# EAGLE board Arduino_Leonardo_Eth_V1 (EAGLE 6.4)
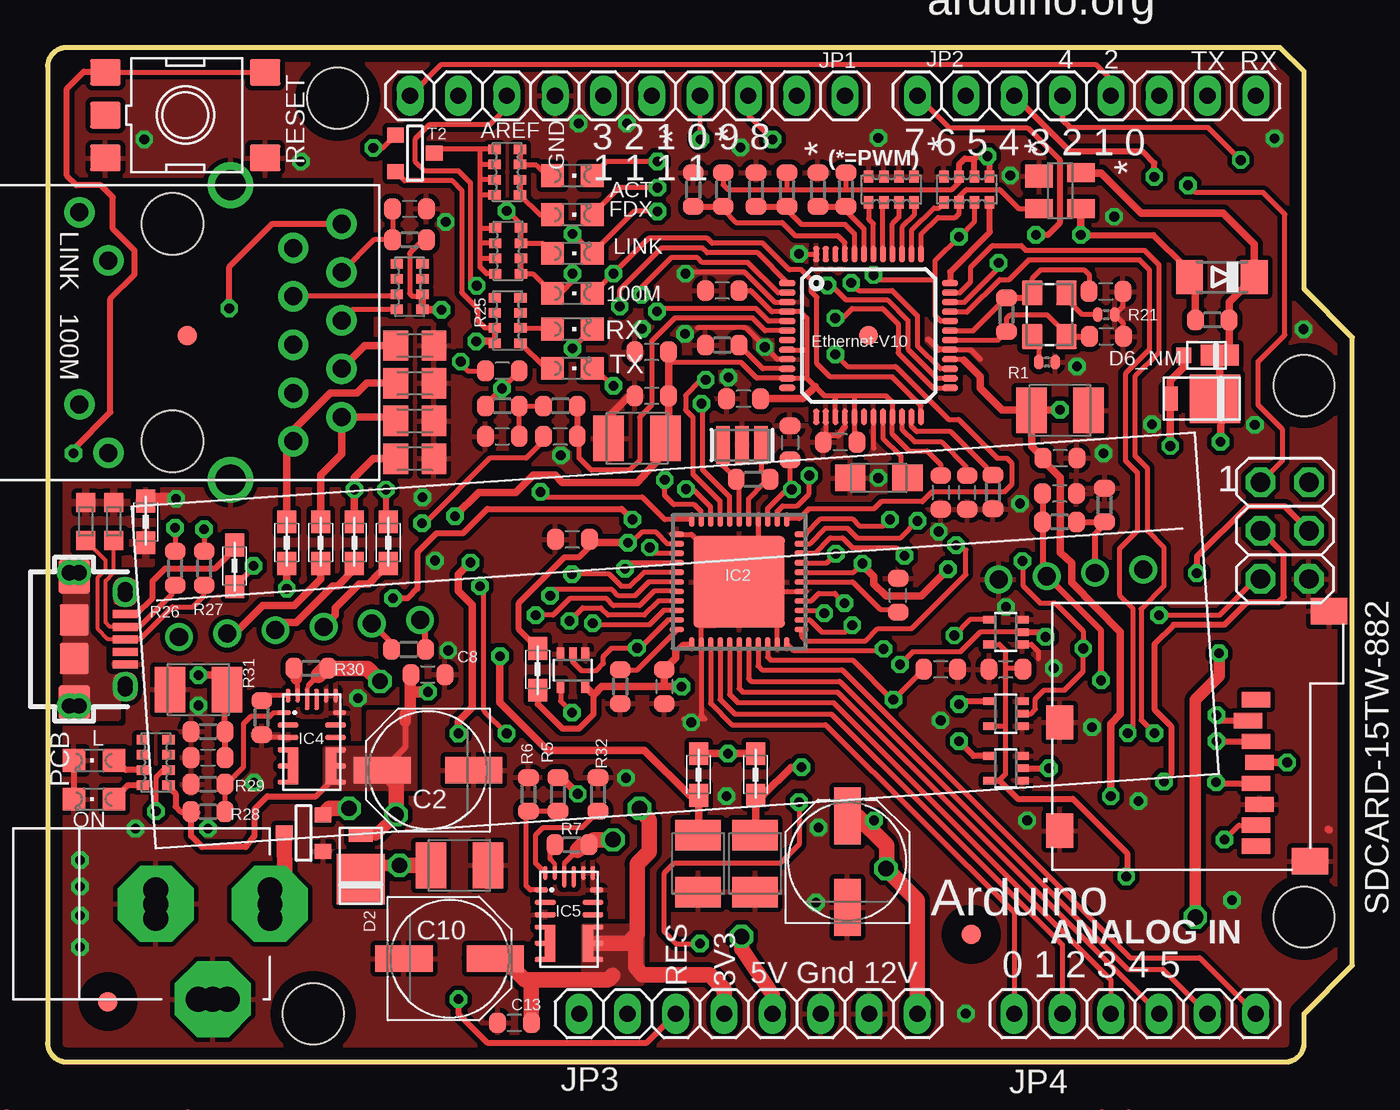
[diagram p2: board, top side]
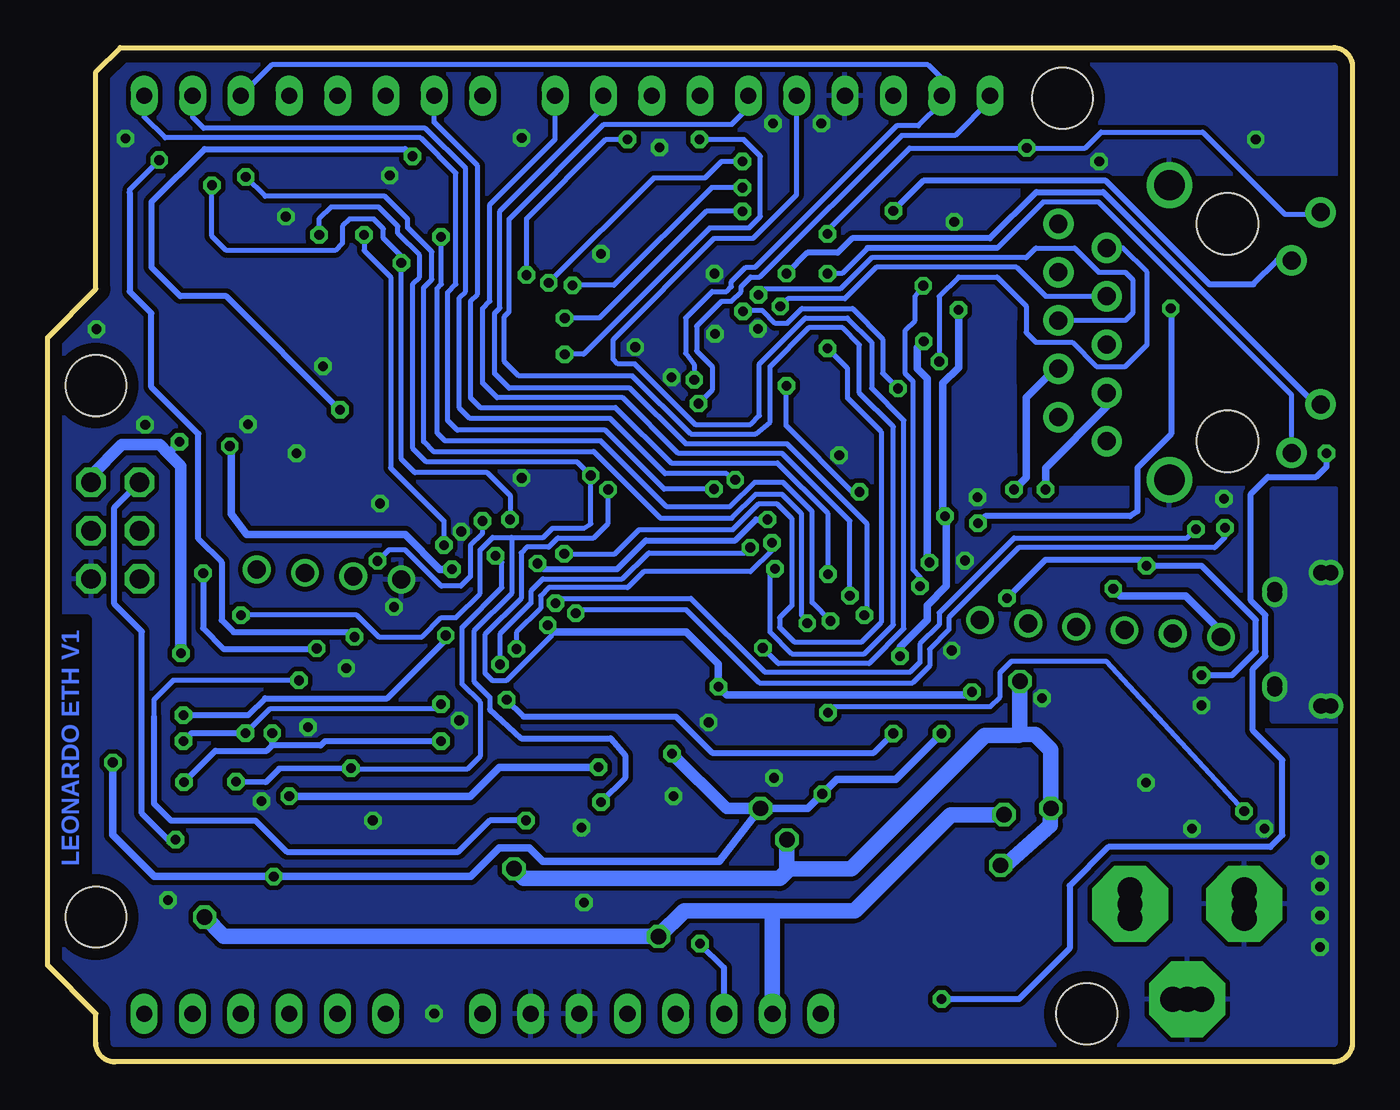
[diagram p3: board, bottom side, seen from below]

Size 68.58 x 53.34 mm. Coordinates in mm from the lower left corner, seen from the top.
Outline: 66.04,2.54 68.58,5.08 68.58,38.1 66.04,40.64 66.04,52.07 64.77,53.34 1,53.34 arc90 0,52.34 0,1 arc90 1,0 65.04,0 arc90 66.04,1 66.04,2.54
Copper layers (1*16): Top 0.035mm / dielectric 1.5mm / Bottom 0.035mm
Design rules "default *": minimum track width 10mil, minimum drill 20mil, track to track 8mil, track to pad 8mil, pad to pad 4mil, via to via 8mil, smd to smd 4mil, copper to edge 25mil, drill to drill 10mil, minimum pad ring 10mil, minimum via ring 8mil, stop-mask expansion 1mil, vias tented up to drill 33mil, thermal gap 10mil
Net classes: 0 default: width 0.254 mm, drill 0.508 mm, clearance 0.102 mm; 1 power: width 0.254 mm, drill 0.508 mm, clearance 0.203 mm; 2 gnd: width 0.254 mm, drill 0.508 mm, clearance 0.254 mm; 3 usbvcc: width 0.254 mm, drill 0.508 mm, clearance 0.254 mm; 4 aref: width 0.254 mm, drill 0.508 mm, clearance 0.203 mm; 5 ETH: width 0.305 mm, drill 0.508 mm, clearance 0.762 mm to class 0, clearance 0.762 mm to class 1, clearance 0.762 mm to class 2, clearance 0.762 mm to class 3, clearance 0.762 mm to class 4
Holes 3.2 mm at 66.04,35.56 66.04,7.62 15.24,50.67 13.97,2.54
bRestrict: 3 lines

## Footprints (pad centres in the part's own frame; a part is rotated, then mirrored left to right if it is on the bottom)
CHIPLED_0805 = smd 1.2 x 1.2: A 0,-1.05; C 0,1.05
C0603-ROUND = smd 0.898 x 1.1: 1 -0.889,0; 2 0.889,0
PANASONIC_D = smd 3 x 1.4: + 2.4,0; - -2.4,0
C0805K = smd 1.3 x 1.6: 1 -1,0; 2 1,0
SMC_B = smd 1.6 x 2.4: + -1.5,0; - 1.5,0
SMC_A = smd 1.6 x 1.4: + -1.5,0; - 1.5,0
DO220AAL = smd 2.667 x 2.54: P$1 -0.7,0 | smd 0.762 x 1.27: P$2 1.65,0
MINIMELF = smd 1.4 x 1.8: A 1.7,0; C -1.7,0
MICROSMP = smd 0.8 x 0.8: A 1.2,0 | smd 2 x 1.1: K -0.7,0
SOT143 = smd 1.2 x 1.44: 1 -0.75,-1.1 | smd 1 x 1.44: 2 0.95,-1.1; 3 0.95,1.1; 4 -0.95,1.1
QFN44ML7X7 = smd 0.75 x 0.3: 1 -3.275,2.5; 2 -3.275,2; 3 -3.275,1.5; 4 -3.275,1; 5 -3.275,0.5; 6 -3.275,0; 7 -3.275,-0.5; 8 -3.275,-1; 9 -3.275,-1.5; 10 -3.275,-2; 11 -3.275,-2.5; 23 3.275,-2.5; 24 3.275,-2; 25 3.275,-1.5; 26 3.275,-1; 27 3.275,-0.5; 28 3.275,0; 29 3.275,0.5; 30 3.275,1; 31 3.275,1.5; 32 3.275,2; 33 3.275,2.5 | smd 0.3 x 0.75: 12 -2.5,-3.275; 13 -2,-3.275; 14 -1.5,-3.275; 15 -1,-3.275; 16 -0.5,-3.275; 17 0,-3.275; 18 0.5,-3.275; 19 1,-3.275; 20 1.5,-3.275; 21 2,-3.275; 22 2.5,-3.275; 34 2.5,3.275; 35 2,3.275; 36 1.5,3.275; 37 1,3.275; 38 0.5,3.275; 39 0,3.275; 40 -0.5,3.275; 41 -1,3.275; 42 -1.5,3.275; 43 -2,3.275; 44 -2.5,3.275 | smd 4.826 x 4.826: EXP 0,0
SC70-5 = smd 0.4 x 0.7: 1 -0.65,-0.85; 2 0,-0.85; 3 0.65,-0.85; 4 0.65,0.85; 5 -0.65,0.85
QFN-20 = smd 0.7 x 0.25: 1 -1.45,1.55; 4 -1.45,-0.4; 5 -1.45,-1.25; 6 -1.45,-2.1; 7 1.45,-2.1; 8 1.45,-1.25; 9 1.45,-0.4; 12 1.45,1.55 | smd 1.1 x 0.25: 2 -1.25,0.9; 3 -1.25,0.25; 10 1.25,0.25; 11 1.25,0.9 | smd 0.25 x 0.7: 13 1.25,2.45; 14 0.75,2.45; 17 -0.75,2.45; 18 -1.25,2.45 | smd 0.25 x 1.1: 15 0.25,2.25; 16 -0.25,2.25 | smd 0.6 x 1.95: 19 -1,-1.25; 20 1,-1.25
TQFP48-7X7 = smd 0.85 x 0.32: 1 -4.275,2.75; 2 -4.275,2.25; 3 -4.275,1.75; 4 -4.275,1.25; 5 -4.275,0.75; 6 -4.275,0.25; 7 -4.275,-0.25; 8 -4.275,-0.75; 9 -4.275,-1.25; 10 -4.275,-1.75; 11 -4.275,-2.25; 12 -4.275,-2.75; 25 4.275,-2.75; 26 4.275,-2.25; 27 4.275,-1.75; 28 4.275,-1.25; 29 4.275,-0.75; 30 4.275,-0.25; 31 4.275,0.25; 32 4.275,0.75; 33 4.275,1.25; 34 4.275,1.75; 35 4.275,2.25; 36 4.275,2.75 | smd 0.32 x 0.85: 13 -2.75,-4.275; 14 -2.25,-4.275; 15 -1.75,-4.275; 16 -1.25,-4.275; 17 -0.75,-4.275; 18 -0.25,-4.275; 19 0.25,-4.275; 20 0.75,-4.275; 21 1.25,-4.275; 22 1.75,-4.275; 23 2.25,-4.275; 24 2.75,-4.275; 37 2.75,4.275; 38 2.25,4.275; 39 1.75,4.275; 40 1.25,4.275; 41 0.75,4.275; 42 0.25,4.275; 43 -0.25,4.275; 44 -0.75,4.275; 45 -1.25,4.275; 46 -1.75,4.275; 47 -2.25,4.275; 48 -2.75,4.275 | smd 1 x 1: P$1 0,0
2X03 = drill 1.016 pad 1.55 octagon: 1 -2.54,-1.27; 2 -2.54,1.27; 3 0,-1.27; 4 0,1.27; 5 2.54,-1.27; 6 2.54,1.27
POWERSUPPLY_DC-21MM = drill 1.3 pad 4 octagon: 1 -5.08,-3.353; 2 -0.076,-6.35; 3 -0.076,-0.356 | drill 1.3: 4 -5.08,-4.115; 5 -5.08,-2.591; 6 -0.838,-0.356; 7 0.686,-0.356; 8 -0.838,-6.35; 9 0.686,-6.35
1X10 = drill 0.85 pad 1.422 long: 1 -11.43,0; 2 -8.89,0; 3 -6.35,0; 4 -3.81,0; 5 -1.27,0; 6 1.27,0; 7 3.81,0; 8 6.35,0; 9 8.89,0; 10 11.43,0
1X08 = drill 0.85 pad 1.422 long: 1 -8.89,0; 2 -6.35,0; 3 -3.81,0; 4 -1.27,0; 5 1.27,0; 6 3.81,0; 7 6.35,0; 8 8.89,0
1X06 = drill 0.85 pad 1.422 long: 1 -6.35,0; 2 -3.81,0; 3 -1.27,0; 4 1.27,0; 5 3.81,0; 6 6.35,0
0805 = smd 1.2 x 1: 1 -1.1,0; 2 1.1,0
CRYSTAL3.2X2.5 = smd 1.3 x 1.1: 1 -1.15,-0.9; 2 1.15,-0.9; 3 1.15,0.9; 4 -1.15,0.9
R0402 = smd 0.508 x 0.762: 1 -0.445,0; 2 0.445,0
R0603-ROUND = smd 0.898 x 1.1: 1 -0.889,0; 2 0.889,0
CAY16 = smd 0.5 x 0.65: 1 -1.2,-0.675; 2 -0.4,-0.675; 3 0.4,-0.675; 4 1.2,-0.675; 5 1.2,0.675; 6 0.4,0.675; 7 -0.4,0.675; 8 -1.2,0.675
TS42 = smd 1.6 x 1.4: 1 -4.2,2.25; 2 4.2,2.25; 3 -4.2,-2.25; 4 4.2,-2.25; 5 -4.2,0
SOT-23 = smd 0.787 x 0.889: 1 0.025,-1.016; 2 -0.94,1.016; 3 0.991,1.016
FIDUCIA-MOUNT = smd 1.016 x 1.016: P$1 0,0
POE-RJ45 = drill 1.6: CH1 13.94,7.75; CH2 13.94,-7.75 | drill 0.95 pad 1.6: L1 7.51,-6.325; L2 5.99,-3.785; L3 7.51,3.785; L4 5.99,6.325; R1 19.77,5.715; R2 17.23,4.445; R3 19.77,3.175; R4 17.23,1.905; R5 19.77,0.635; R6 17.23,-0.635; R7 19.77,-1.905; R8 17.23,-3.175; R9 19.77,-4.445; R10 17.23,-5.715 | hole 3.25: 10.89,5.715; 10.89,-5.715
CON2_USB_MICRO_B_AT = smd 0.406 x 1.346: P1 -1.321,2.692; P2 -0.66,2.692; P3 0,2.692; P4 0.66,2.692; P5 1.321,2.692 | drill 0.8 pad 1.24: P$1 -2.616,2.692; P$2 -2.362,2.692; P$7 2.362,2.692; P$8 2.616,2.692 | drill 0.8 pad 1.25: P$3 -3.505,-0.254; P$4 -3.505,0.254; P$5 3.505,0.254; P$6 3.505,-0.254 | smd 1.778 x 1.651: S1 -3.302,0; S2 3.302,0 | smd 1.524 x 1.27: S3 -2.489,2.692; S4 2.489,2.692 | smd 1.626 x 1.524: S5 -1.016,0; S6 1.016,0
SDCARD-15TW-8821 = smd 0.8 x 1.5: 1 0,0; 2 1.1,-0.4; 3 2.2,0; 4 3.3,0.2; 5 4.4,0; 6 5.5,0.2; 7 6.6,0; 8 7.7,0 | smd 1.4 x 1.9: GND1 -4.66,3.85; GND2 8.49,2.85 | smd 1.8 x 1.4: GND3 1.19,-10.3; GND4 6.89,-10.3
RESONATOR = smd 0.7 x 2: 1 -1,0; 2 0,0; 3 1,0
CT/CN0603 = smd 1 x 1: 1 -1,0; 2 1,0
AG9000 = drill 0.95 pad 1.422: P$1 0,0; P$2 2.54,0; P$3 5.08,0; P$4 7.62,0; P$5 10.16,0; P$6 12.7,0; P$7 43.18,0; P$8 45.72,0; P$9 48.26,0; P$10 50.8,0

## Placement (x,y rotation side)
100M  Green  [CHIPLED_0805]  27.58,40.41 270 top
ACT  Green  [CHIPLED_0805]  27.58,46.61 270 top
C1  100nF  [C0603-ROUND]  19.02,44.86 180 top
C2  47uF  [PANASONIC_D]  19.99,15.34 180 top
C3  10pF  [C0603-ROUND]  55.63,40.51 0 top
C4  10nF  [C0603-ROUND]  23.9,32.89 0 top
C5  10pF  [C0603-ROUND]  55.65,38.15 0 top
C6  10nF  [C0603-ROUND]  26.95,32.89 180 top
C7  10nF  [C0603-ROUND]  23.9,36.35 180 top
C8  100nF  [C0603-ROUND]  19.99,20.37 0 top
C9  10nF  [C0805K]  19.3,35.69 180 top
C10  47uF  [PANASONIC_D]  21.13,5.44 0 top
C11  22uF  [SMC_B]  21.64,10.34 0 top
C12  10nF  [C0805K]  19.3,33.71 180 top
C13  100nF  [C0603-ROUND]  24.54,2.06 180 top
C14  47uF  [PANASONIC_D]  42.04,10.54 90 top
C15  1uF  [C0603-ROUND]  53.19,29.9 180 top
C22  1uF  [C0603-ROUND]  50.37,20.65 180 top
C23  10nF  [C0805K]  19.3,31.72 180 top
C24  100nF  [C0603-ROUND]  46.94,20.65 180 top
C25  1uF  [C0603-ROUND]  44.7,24.54 90 top
C26  1uF  [C0603-ROUND]  27.58,27.48 180 top
C27  100nF  [C0603-ROUND]  39.01,32.56 270 top
C28  100nF  [C0603-ROUND]  32.41,19.74 270 top
C29  10nF  [C0805K]  19.3,37.67 180 top
C31  22uF  [SMC_B]  7.92,19.58 180 top
C32  100nF  [C0603-ROUND]  8.43,16 0 top
C33  22uF  [SMC_B]  53.21,34.26 0 top
C34  100nF  [C0603-ROUND]  53.21,31.75 180 top
C36  10nF  [C0603-ROUND]  48.34,29.95 90 top
C37  22uF  [SMC_B]  37.19,10.44 270 top
C38  22uF  [SMC_B]  34.19,10.44 270 top
C39  100nF  [C0603-ROUND]  35.46,40.56 180 top
C40  100nF  [C0603-ROUND]  46.94,29.95 270 top
C41  100nF  [C0603-ROUND]  41.66,32.59 180 top
C42  100nF  [C0603-ROUND]  31.75,35.03 180 top
C43  100nF  [C0603-ROUND]  36.58,34.87 180 top
C44  22uF  [SMC_B]  30.99,32.79 180 top
C45  100nF  [C0603-ROUND]  31.75,37.34 180 top
C46  4u7  [SMC_A]  43.69,30.71 180 top
D1  SS1P3L  [DO220AAL]  60.66,34.87 180 top
D2  SS1P3L  [DO220AAL]  16.46,10.31 90 top
D4  CD1206-S01575  [MINIMELF]  61.72,41.27 180 top
D6_NM  MSS1P3L-M3/89A  [MICROSMP]  60.91,37.16 180 top
FDX  Yellow  [CHIPLED_0805]  27.58,44.55 270 top
IC1  CAT811TTBI-CT3  [SOT143]  53.21,45.82 270 top
IC2  ATMEGA32U4-MUR  [QFN44ML7X7]  36.35,25.25 180 top
IC3  SN74LVC1G125DCKR  [SC70-5]  27.61,20.6 180 top
IC4  MPM3610  [QFN-20]  13.89,16.81 0 top
IC5  MPM3610  [QFN-20]  27.41,7.49 0 top
IC6  0982_W5500  [TQFP48-7X7]  43.15,38.2 0 top
IC10  SN74LVC1G125DCKR  [SC70-5]  50.37,18.31 90 top
IC11  SN74LVC1G125DCKR  [SC70-5]  50.37,15.44 90 top
IC12  SN74LVC1G125DCKR  [SC70-5]  50.37,22.61 90 top
ICSP  ICSP  [2X03]  65.02,27.94 270 top
JK1  POWER-SUPPLY  [POWERSUPPLY_DC-21MM]  5.33,8.38 90 top
JP1  FH254-110DF08500T30  [1X10]  30.48,50.8 180 top
JP2  FH254-108DF08500T20  [1X08]  54.61,50.8 180 top
JP3  FH254-108DF08500T21  [1X08]  36.83,2.54 0 top
JP4  FH254-106DF08500T10  [1X06]  57.15,2.54 0 top
L  Green  [CHIPLED_0805]  2.44,15.85 90 top
L1  10uH  [0805]  25.76,20.65 90 top
L3  MH2029-300Y  [0805]  37.21,15.11 270 top
L5  MH2029-300Y  [0805]  9.83,26.09 90 top
L6  MH2029-300Y  [0805]  5.16,28.4 270 top
L7  MH2029-300Y  [0805]  12.57,27.3 270 top
L8  MH2029-300Y  [0805]  14.35,27.3 270 top
L9  MH2029-300Y  [0805]  17.91,27.3 270 top
L10  MH2029-300Y  [0805]  16.13,27.3 270 top
L12  MH2029-300Y  [0805]  34.21,15.11 270 top
LINK  Yellow  [CHIPLED_0805]  27.58,42.52 270 top
ON  Green  [CHIPLED_0805]  2.44,13.82 90 top
Q4  FTX25.000M12SM3S  [CRYSTAL3.2X2.5]  52.65,39.29 270 top
R1  0R  [R0402]  52.53,36.8 180 top
R2  10k  [R0603-ROUND]  49.68,29.97 90 top
R3  12k4_1%  [R0603-ROUND]  35.46,37.69 0 top
R4  10k  [R0603-ROUND]  35.51,45.87 90 top
R5  75K  [R0603-ROUND]  26.82,14.07 90 top
R6  24K_0.1%  [R0603-ROUND]  25.27,14.07 270 top
R7  100k  [R0603-ROUND]  27.56,11.43 180 top
R8  0R  [R0603-ROUND]  53.19,28.4 0 top
R9  NM  [R0603-ROUND]  18.97,21.69 0 top
R10  NM  [R0603-ROUND]  55.55,29.29 90 top
R11  10k  [R0603-ROUND]  33.93,45.87 270 top
R12  10k  [R0603-ROUND]  38.86,45.87 90 top
R13  1M  [R0603-ROUND]  37.08,30.63 0 top
R14  1M  [R0603-ROUND]  50.39,39.29 270 top
R15  10k  [R0603-ROUND]  37.24,45.87 270 top
R16  10k  [R0603-ROUND]  61.21,39.01 0 top
R17  10k  [R0603-ROUND]  30.1,19.74 90 top
R18  10k  [R0603-ROUND]  8.43,17.37 0 top
R19  10k  [R0603-ROUND]  41.96,45.87 90 top
R20  10k  [R0603-ROUND]  40.49,45.87 270 top
R21  0R  [R0402]  55.65,39.29 0 top
R22  100R_1%  [R0603-ROUND]  23.9,34.49 180 top
R23  100R_1%  [R0603-ROUND]  26.95,34.49 0 top
R24  22R  [R0603-ROUND]  19.02,43.23 180 top
R25  1K  [CAY16]  24.18,38.99 90 top
R26  22R  [R0603-ROUND]  6.71,25.96 90 top
R27  22R  [R0603-ROUND]  8.23,25.96 90 top
R28  100K_1%  [R0603-ROUND]  8.43,13.16 180 top
R29  19K1_0.1%  [R0603-ROUND]  8.43,14.61 0 top
R30  100k  [R0603-ROUND]  13.84,20.7 180 top
R31  56k  [R0603-ROUND]  11.25,18.11 90 top
R32  39K  [R0603-ROUND]  28.93,14.07 270 top
RESET  TS42  [TS42]  7.24,49.78 0 top
RN1  1K  [CAY16]  5.69,15.75 90 top
RN2  49R9  [CAY16]  19.02,40.77 90 top
RN3  1K  [CAY16]  24.21,42.65 270 top
RN4  1K  [CAY16]  24.16,46.79 270 top
RN8  10k  [CAY16]  48.31,45.87 0 top
RN9  10k  [CAY16]  44.35,45.87 0 top
RX  Yellow  [CHIPLED_0805]  27.58,38.53 270 top
T1  PMV48XP  [SOT-23]  13.46,12.06 270 top
T2  PMV48XP  [SOT-23]  19.3,47.75 90 top
TX  Yellow  [CHIPLED_0805]  27.58,36.47 270 top
U$1  DISCLAIMER  [DISCLAIMER]  not placed on the board
U$2  FIDUCIALMOUNT  [FIDUCIA-MOUNT]  7.34,38.2 0 top
U$4  FIDUCIALMOUNT  [FIDUCIA-MOUNT]  48.54,6.71 0 top
U$5  FIDUCIALMOUNT  [FIDUCIA-MOUNT]  3.17,3.17 0 top
UC1  RB1-125BHQ1A  [POE-RJ45]  -4.32,38.35 0 top
USB1  MCR-B-S-RA-SMT-CS1TR  [CON2_USB_MICRO_B_AT]  1.4,22.23 270 top
X2  SDCARD-15TW-882  [SDCARD-15TW-8821]  63.5,19.05 270 top
Y1  CSTCE16M0V53-R0  [RESONATOR]  36.5,32.44 0 top
Z1  BRNCG0603MLC-05E  [CT/CN0603]  2.01,28.42 90 top
Z2  BRNCG0603MLC-05E  [CT/CN0603]  3.48,28.42 90 top
ZZ1  AG9612-2BR  [AG9000]  6.91,22.35 4 top

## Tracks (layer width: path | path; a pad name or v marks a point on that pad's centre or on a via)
1V2O
  Top 0.254: 48.26,30.76 48.26,31.32 46.97,32.61 45.57,32.61 44.91,33.28 IC6.22
  Top 0.305: 48.26,30.76 C36.2
3V3_LED
  Top 0.254: 23.51,41.55 RN3.4 23.07,41.45 22.73,41.78 22.73,42.29 | RN3.1 23.53,43.83 | 23.53,43.83 23.52,43.94 | 22.73,42.29 22.73,43.18 | 22.73,43.18 22.73,43.94 | 22.73,43.94 22.73,45.59 | 22.73,45.59 22.73,46.35 | 22.73,46.35 22.73,47.12 | 22.73,47.12 22.73,47.99 | 23.46,48.01 RN4.1 22.73,47.99 | 22.73,47.99 20.53,47.99 T2.1 | RN4.2 22.8,47.19 22.73,47.12 | RN4.3 22.77,46.39 22.73,46.35 | RN4.4 22.74,45.59 22.73,45.59 | 23.53,43.83 22.74,43.83 22.73,43.94 | RN3.2 22.74,43.05 22.73,43.18 | RN3.3 22.78,42.25 22.73,42.29
+3V3  (via drill 0.51, 0.81)
  Top 0.254: T2.2 18.77,46.33 21.29,46.33 21.77,45.85 21.77,40.46 22.61,39.62 22.61,38.99 22.99,38.61 23.49,38.61 R25.7 | IC12.5 50.03,21.96 50.34,21.64 50.34,20.7 | 49.53,17.68 IC10.5 50.33,17.66 50.34,17.65 | 50.34,20.7 50.34,17.65 | 50.34,17.65 50.34,15.11 50.03,14.79 | C22.1 51.21,20.7 50.34,20.7
  Top 0.305: 64.26,15.75 X2.4 | v56.69,9.75 56.74,9.8 56.74,10.97 53.87,13.84 50.98,13.84 50.03,14.79 IC11.5 49.9,14.79 | 49.4,21.95 IC12.5 | R25.7 R25.8 23.49,37.9
  Top 0.406: v65.15,15.75 64.26,15.75 | v22.53,37.9 23.49,37.9 | v22.23,26.26 21.59,25.63 21.59,24.77 22.33,24.03 22.33,18.64 21.59,17.91 v21.59,17.27 | R5.2 27,14.96 v27.86,14.1 | L12.1 v35.76,16.21 | v35.76,16.21 v35.76,16.2 | v35.76,16.21 L3.1
  Top 0.813: JP3.4 35.56,3.81 34.8,4.57 31.24,4.57 30.92,5.02 30.92,6.67 | 29.7,4.56 29.46,4.32 25.65,4.32 | 25.65,4.32 25.07,4.32 23.9,5.49 23.88,5.46 22.41,5.46 C10.+ | C13.1 25.43,4.29 25.65,4.32 | 30.92,6.67 30.99,6.73 30.99,10.41 31.62,11.05 31.62,12.7 v31.11,13.34 | 30.92,6.67 30.5,6.24 IC5.8
  Bottom 0.406: v21.59,17.27 24,14.86 27.1,14.86 v27.86,14.1 28.63,13.34 v31.11,13.34 33.27,10.54 42.55,10.54 43.26,11.25 44.83,11.25 46.33,9.75 v56.69,9.75 62.97,9.75 65.15,11.94 v65.15,15.75 | v22.53,37.9 22.86,37.57 22.86,36.45 22.35,35.94 22.35,26.39 v22.23,26.26
  Bottom 0.61: v35.76,16.2 32.89,13.34 v31.11,13.34
  pour Top (no thermals): 31.24,7.11 28.17,7.11 28.17,4.17 31.24,4.17
+3V3A  (via drill 0.51)
  Top 0.254: 38.87,37.44 IC6.8 38.89,37.44 39.75,37.44 39.9,37.47 | 42.42,35.03 44.07,35.03 44.4,34.7 IC6.21 44.41,33.02 45.29,32.13 46.23,32.13 46.94,31.42 C40.1 | 42.42,35.03 41.4,35.03 | 41.4,35.03 40.84,35.03 40.35,35.52 39.9,35.97 | IC6.15 41.41,34.85 41.4,34.85 41.4,35.03 | 39.9,37.47 39.9,39.12 39.57,39.45 IC6.4 38.07,39.45 36.96,40.56 C39.1 | 39.9,37.47 39.9,35.97 | 42.42,35.03 42.42,33.94 IC6.17 42.42,33.91 42.42,33.15 42.55,33.02 C41.1 | 39.9,35.97 39.89,35.95 IC6.11 37.28,35.95 36.45,36.78 32.69,36.78 32.64,36.83 | R24.1 19.48,42.98 19.02,42.52 19.02,40.41 19.18,40.26 19.68,40.26 RN2.2 19.53,40.24
  Top 0.406: C43.1 39.7,34.87 40.35,35.52 | RN2.2 RN2.1 20.68,39.57 v20.7,39.55 | v23.77,21.34 23.77,18.9 26.29,16.38 31.37,16.38 33.74,14.01 L12.2 34.21,11.94 C38.+ | v21.41,28.7 22.66,29.95 24.61,29.95 25.53,30.86 26.67,30.86 27.05,30.48 30.99,30.48 32.38,32 32.38,32.69 C44.+ 32.64,32.94 C42.1 32.64,36.83 C45.1
  Bottom 0.406: v20.7,39.55 20.7,36.52 21.54,35.69 21.54,28.83 v21.41,28.7 21.34,28.5 21.34,25.02 22.35,24 22.35,23.24 23.77,21.82 v23.77,21.34
+3V3D  (via drill 0.51)
  Top 0.254: R4.2 35.51,46.13 35.76,45.87 38.86,45.87 | 38.86,45.87 41.96,45.87 | 41.96,45.87 47.52,45.87 47.91,46.26 RN8.7 | R12.2 38.86,45.87 | R19.2 41.96,45.87 | 51.69,34.29 C33.+ | IC6.28 48.14,36.95
  Top 0.305: RN8.7 47.91,47.2 48.21,47.5 48.72,47.5 | 49.53,46.52 RN8.5 49.51,47.52 v49.4,47.62 48.84,47.62 48.72,47.5 | RN8.6 48.71,47.49 48.72,47.5 | C34.2 52.32,31.62 | 51.74,34.29 C33.+ | 48.14,36.95 48.16,36.9
  Top 0.406: 48.16,36.9 49.02,36.04 49.02,35.43 50.16,34.29 51.69,34.29 | C33.+ 51.71,32.36 C34.2 | 52.32,31.62 53.21,30.73 53.21,26.8 53.82,26.24 53.82,25.22 56.39,22.61 56.39,18.29 55.88,17.78 v55.88,13.97 | v53.21,34.29 51.74,34.29 | v39.62,15.49 39.07,15.49 37.59,14.01 L3.2 37.21,11.96 C37.+
  Bottom 0.305: v53.21,34.29 59.18,40.26 61.59,40.26 63.12,41.78 63.12,45.21 60.33,48.01 49.78,48.01 v49.4,47.62
  Bottom 0.406: v55.88,13.97 46.35,13.97 44.83,15.49 v39.62,15.49
+5V  (via drill 0.51, 0.81)
  Top 0.254: IC2.2 40.05,23.25 40.69,22.61 41.94,22.61 v42.29,22.96 | IC2.34 33.83,21.96 33.39,21.96 33.02,21.59 | IC2.14 37.85,29.11 38.84,30.1 v39.12,30.1 39.01,30.2 C27.2
  Top 0.305: IC4.8 IC4.20 | 7.87,13.11 R28.2 | 54.95,46.77 IC1.4 54.32,46.76 | IC4.7 14.84,14.71 14.1,13.97 11.56,13.97 10.87,13.28 10.87,11.89 10.41,11.3 8.13,11.3 7.54,11.89 R28.2 | 18.8,17.91 18.8,16.55 C2.+ | RN1.1 6.37,14.46 6.73,14.1 6.73,13.44 7.01,13.16 R28.2 | L1.1 25.76,18.82 27.05,17.53 27.94,17.53 28.7,18.29 28.7,19.31 | 32.41,19.76 32.38,19.74
  Top 0.406: IC3.5 28.7,19.31 29.13,19.74 32.38,19.74 v33.33,19.74 | v61.65,32.61 61.71,34.46 D1.P$1 61.61,35.13 D6_NM.K 62.1,37.65 R16.2 62.1,39.96 D4.C 63.42,43 61.8,44.63 57.48,44.63 55.37,46.74 54.99,46.74 54.95,46.77 | 19.07,20.34 C8.1 | 32.41,19.76 C28.1 33.02,21.23 33.02,21.59
  Top 0.61: v61.57,21.49 61.57,20.3 60.33,19.05 v60.33,7.62 | D2.P$2 17.25,11.94 v18.31,13.01 | 18.8,17.91 18.8,18.29 19.05,18.54 19.05,19.43 | 19.05,19.43 19.05,20.32 C8.1 | v19.99,19.46 19.07,19.46 19.05,19.43
  Top 0.813: v18.31,13.01 18.31,14.62 C2.+ | v36.47,6.6 36.47,5.94 38.1,3.56 JP3.5
  Bottom 0.254: v42.29,22.96 42.06,22.45 44.45,20.07 45.21,20.07 45.59,20.45 45.59,22.48 43.69,24.38 43.69,26.77 43.41,27.08 42.24,27.08 41.76,27.56 39.88,27.56 39.12,28.32 v39.12,30.1
  Bottom 0.406: v42.29,22.96 41.94,22.61 35,22.61 33.33,20.93 v33.33,19.74 32.89,19.3 20.19,19.3 v19.99,19.46 | v61.65,32.61 61.65,32.59 62.23,32
  Bottom 0.61: v61.57,21.49 61.57,31.34 62.23,32 62.69,32.46 64.67,32.46 66.29,30.84 ICSP.2
  Bottom 0.813: 30.48,7.95 26.16,7.95 21.11,13.01 v18.31,13.01 | v60.33,7.62 59.31,6.6 v36.47,6.6 35.13,7.95 30.48,7.95 | JP3.2 30.48,7.95
  pour Top (no thermals): 14.61,16.51 16.89,16.51 16.89,18.41 19.3,18.41 19.3,14.35 14.61,14.35
A0
  Top 0.254: IC2.36 34.85,18.85 35.97,17.73 40.89,17.73 50.8,7.87 JP4.1
A1
  Top 0.254: IC2.37 35.35,19.06 36.12,18.29 41.2,18.29 53.34,6.17 JP4.2
A2
  Top 0.254: IC2.38 35.85,19.32 36.27,18.9 41.3,18.9 55.88,4.32 JP4.3
A3
  Top 0.254: IC2.39 36.35,19.63 36.52,19.46 41.5,19.46 JP4.4
A4
  Top 0.254: IC2.40 36.85,20.15 36.98,20.02 41.63,20.02 56.77,4.88 58.62,4.88 JP4.5
A5
  Top 0.254: IC2.41 37.35,20.82 37.54,20.62 41.76,20.62 56.9,5.49 60.55,5.49 JP4.6
ACT  (via drill 0.51)
  Top 0.254: v42.24,40.97 42.62,40.56 44.4,40.56 45.72,39.24 45.72,37.67 46.94,36.45 IC6.27 | v32.05,47.35 29.37,47.35 ACT.C
  Bottom 0.254: v42.24,40.97 36.73,46.48 34.04,46.48 33.17,47.35 v32.05,47.35
AREF  (via drill 0.51)
  Top 0.254: IC2.42 37.85,21.28 38,21.13 42.32,21.13 44.4,19.05 v44.45,19.05 C24.2 45.8,20.52 | JP1.8 24.13,50.16 23.24,49.28 20.07,49.28 19.3,48.51 19.3,47.37 19.81,46.86 21.59,46.86 22.23,46.23 22.23,41.02 v22.55,40.82 | v22.73,25.02 22.94,24.82 22.94,18.47 v24.13,17.27
  Bottom 0.254: v22.55,40.82 22.99,40.26 22.99,38.99 23.5,38.48 23.5,36.2 23.09,35.79 23.09,25.88 22.73,25.53 v22.73,25.02
  Bottom 0.305: v44.45,19.05 43.56,18.16 35.56,18.16 33.66,16.26 25.15,16.26 v24.13,17.27
AVCC  (via drill 0.51)
  Top 0.254: IC2.44 39.18,21.64 43.87,21.64 v43.94,21.72 | IC2.24 32.59,27.25 31.98,27.86 31.24,27.86 30.68,27.3 v30.5,27.3
  Top 0.305: L1.2 24.77,22.74 24.77,24.13 27.18,26.54 27.94,26.54 28.65,27.25 C26.1
  Top 0.406: C26.1 28.96,27.3 v30.5,27.3
  Bottom 0.254: v30.5,27.3 30.5,26.92 31.65,25.78 37.24,25.78 38.1,24.94 42.24,24.94 42.67,24.51 42.67,23.85 43.94,22.58 v43.94,21.72
D0/RX  (via drill 0.51)
  Top 0.254: IC2.20 34.85,29.19 33.91,30.12 v33.55,30.12
  Bottom 0.254: v33.55,30.12 36.17,30.12 39.27,33.22 47.04,33.22 47.55,33.73 47.55,40.46 47.12,40.89 47.12,46.74 48.97,48.59 62.41,48.59 63.5,49.68 JP2.1
D1/TX  (via drill 0.51)
  Top 0.254: IC2.21 34.35,28.95 33.98,29.31 32.92,29.31 32.44,29.79 v32.44,30.61
  Bottom 0.254: JP2.2 60.96,49.68 60.38,49.1 48.72,49.1 46.61,46.99 46.61,40.51 46.94,40.18 46.94,34.39 46.38,33.83 39.01,33.83 36.12,30.94 32.89,30.94 v32.44,30.61
D2/SDA  (via drill 0.51)
  Top 0.254: IC2.19 35.35,29.47 33.91,30.91 33.91,33.91 33.53,34.29 33.53,35.05 34.34,35.87 v34.59,35.87
  Bottom 0.254: JP2.3 56.79,52.43 22.3,52.43 21.54,51.66 21.54,50.85 JP1.9 21.59,50.44 22.81,49.23 23.95,49.23 31.39,41.78 31.88,41.78 32.64,41.02 32.64,40.77 32.89,40.51 33.66,40.51 35.05,39.12 35.05,37.26 34.59,36.68 v34.59,35.87
D3/SCL  (via drill 0.51)
  Top 0.254: IC2.18 35.85,29.71 34.42,31.14 34.42,34.57 v34.37,34.62 | JP2.4 55.88,51.66 55.12,52.43 20.68,52.43 JP1.10
  Bottom 0.254: JP1.10 19.05,50.55 20.88,48.72 23.7,48.72 31.14,41.27 31.62,41.27 32.13,40.77 32.13,40.51 32.64,40.01 33.15,40.01 34.47,38.68 34.47,37.39 33.66,36.58 33.66,35.33 v34.37,34.62
D4/SD_CS  (via drill 0.51)
  Top 0.254: IC12.2 49.02,22.61 47.98,21.57 45.47,21.57 v44.81,20.9 | IC2.25 31.95,26.75 v31.65,27.05 | 53.72,49.15 60.98,49.15 v62.71,47.42
  Top 0.305: IC12.2 52.2,22.61 v52.45,22.35 | JP2.5 53.34,49.53 53.72,49.15
  Bottom 0.254: v44.81,20.9 44.81,22.5 43.18,24.13 43.18,24.77 42.55,25.4 38.38,25.4 36.98,26.77 31.93,26.77 v31.65,27.05 | v62.71,47.42 64.26,45.87 64.26,45.72
  Bottom 0.305: v52.45,22.35 52.7,22.61 58.8,22.61 59.44,23.24 59.44,26.29 60.66,27.51 60.66,33.02 63.12,35.48 63.12,39.37 64.26,40.51 64.26,45.72
D5*  (via drill 0.51)
  Top 0.254: v28.65,23.06 28.98,22.99 31.62,22.99 32.38,23.75 IC2.31
  Top 0.305: v58.17,46.53 58.17,47.27 57.56,47.88 53.72,47.88 JP2.6
  Bottom 0.254: v28.65,23.06 28.96,23.5 28.96,28.83 29.97,29.84 31.37,29.84 32.61,28.6 36.37,28.6 39.88,32.11 48.31,32.11 48.82,32.61 48.82,40.72 48.39,41.15 48.39,42.6 49.66,43.87 49.66,44.32 50.85,45.52 57.15,45.52 v58.17,46.53
D6*  (via drill 0.51)
  Top 0.254: v27.56,25.65 29.52,25.65 30.15,25.02 30.61,25.02 31.34,25.75 IC2.27
  Bottom 0.254: JP2.7 48.26,49.4 45.97,47.12 45.97,40.39 46.35,40.01 46.35,34.92 45.85,34.42 38.73,34.42 35.81,31.5 30.23,31.5 27.56,28.83 v27.56,25.65
D7  (via drill 0.51)
  Top 0.254: IC2.1 39.62,22.4 39.88,22.15 43,22.15 43.64,22.78 45.41,22.78 48.26,25.63 48.26,26.92 v47.75,27.18 | 53.19,47.45 51.54,49.1 47.42,49.1 JP2.8
  Top 0.305: v51.94,43.48 52.58,43.48 53.19,44.09 53.19,47.45
  Bottom 0.254: v51.94,43.48 51.94,42.67 50.55,41.27 50.55,31.24 47.75,28.45 v47.75,27.18
D+
  Top 0.203: 4.06,22.25 3.15,22.25 2.64,22.76 2.64,25.48 3.05,25.88 3.05,26.38 Z1.1
  Top 0.254: USB1.P3 4.06,22.25 4.88,22.25 6.55,23.93 7.62,23.93 8.23,24.54 R27.1
D-
  Top 0.203: 4.06,22.91 3.25,22.91 3.05,23.11 3.05,25.3 3.48,25.73 Z2.1
  Top 0.254: USB1.P2 4.06,22.91 4.85,22.91 6.58,24.64 R26.1
FDXLED  (via drill 0.51)
  Top 0.254: v41,40.84 41.2,40.84 41.96,40.08 44.12,40.08 45.21,38.99 45.21,37.49 46.76,35.94 47.42,35.94 IC6.26 | v32.05,45.97 30.06,45.97 FDX.C
  Bottom 0.254: v32.05,45.97 33.68,45.97 38.81,40.84 v41,40.84
GND  (via drill 0.51)
  Top 0.254: 35.78,23.63 35.11,22.96 34.39,22.96 34.35,22.92 IC2.35 34.35,18.23 34.54,18.03 33.43,18.03 | IC2.43 38.35,24.73 38.35,24.74 | 38.35,24.74 IC2.5 | IC6.14 40.91,32.98 | IC2.15 37.35,26.25 36.72,25.62 | 36.72,25.62 IC2.EXP 33.85,27.75 IC2.23 | 38.35,24.74 37.59,24.74 36.72,25.62 | IC12.1 51.7,21.96 52.07,21.59 52.07,21.21 | C3.2 56.52,39.71 R21.2 56.54,38.85 C5.2 | 46.83,37.45 48.53,37.45 49.02,36.96 | 40.39,42.46 39.2,42.46 v39.5,42.49 | IC6.16 41.91,33.4 | v33.53,41.45 33.66,41.53 36.65,41.53 38.23,39.95 IC6.3 | IC4.3 11.41,17.07 R31.1 | IC6.9 38.36,36.95 36.7,38.61 34.16,38.61 | IC6.19 43.41,32.29 43.43,32.26
  Top 0.305: 53.03,18.03 X2.GND3 | L.C ON.C | 35.78,23.63 IC2.EXP | 40.39,42.46 IC6.48 | IC6.29 46.83,37.45 46.28,38 | 40.91,32.98 40.89,32.97 41.6,32.97 41.91,33.4
  Top 0.406: 67.35,12.19 67.3,12.24 | C42.2 30.58,35.03 29.46,33.91 29.46,32.81 C44.-
  Top 0.61: L6.1 5.28,29.62 v6.76,29.62
  other vias: 48.26,2.54 16.31,19.13 62.26,8.51 40.39,8.38 5.08,48.51 51.49,12.7 55.5,32 46.94,17.96 36.42,48.08 43.66,48.59 30.45,49.35 57.33,13.72 54.89,17.6 10.85,14.68 4.62,12.27 27.91,49.35 46.84,27.89 56.06,44.45 58.04,33.53 63.45,33.5 51.1,29.36 52.88,20.7 33.83,17.86 40.51,12.32 64.49,48.56 50.6,46.61 50.37,23.93 54.1,36.58 13.31,47.35 35.79,35.99 20.93,44.17 8.43,12.27 1.7,10.62 1.7,9.22 1.7,7.7 1.7,6.05 30.4,14.94 33.5,38.28 7.92,18.75 20.37,26.37 19.71,29.69 21.06,21.64 66.01,38.53 43.66,30.71 35.69,13.97 26.97,31.9 37.69,37.59 31.24,38.56
  pour Top (isolate 0.254, rank 2): 0.51,30.1 17.27,30.1 17.27,46.61 0,46.61 0,53.21 64.26,52.83 65.53,51.56 65.53,40.13 68.07,37.59 68.07,5.59 65.53,3.05 65.53,1.51 arc-90 64.53,0.51 31.75,0.51 1.51,0.51 arc-90 0.51,1.51
  pour Bottom (isolate 0.254, rank 2): 17.53,46.74 0.38,46.74 0.38,52.96 64.26,52.83 65.53,51.56 65.53,40.13 68.07,37.59 68.07,5.59 65.53,3.05 65.53,1.51 arc-90 64.53,0.51 -0.02,0.36 -0.05,30.15 17.73,30.15 17.78,37.47
HWB
  Top 0.254: 33.06,22.73 IC2.33 | 33.05,22.72 IC2.33 | R17.2 31.03,20.62 31.03,20.64 33.07,22.68 IC2.33
INT
  Top 0.305: RN8.4 49.53,45.13 49.53,43.64 47.43,41.54 IC6.36
IO8  (via drill 0.51)
  Top 0.254: IC2.28 31.6,25.25 30.86,24.51 30,24.51 29.67,24.84 26.59,24.84 v26.42,24.51
  Bottom 0.254: JP1.1 41.91,48.51 45.34,45.09 45.34,40.01 45.72,39.62 45.72,35.69 44.96,34.92 38.35,34.92 35.43,32 29.97,32 26.42,28.45 v26.42,24.51
IO9*  (via drill 0.51)
  Top 0.254: IC2.29 33.05,24.77 31.88,24.77 31.11,24 29.74,24 29.39,24.36 27.43,24.36 26.57,23.5 v25.65,23.5
  Bottom 0.254: JP1.2 39.37,50.16 44.81,44.73 44.81,39.65 45.09,39.37 45.09,36.2 44.32,35.43 37.97,35.43 35.05,32.51 29.72,32.51 25.53,28.32 25.53,23.62 v25.65,23.5
IO10*/SS  (via drill 0.51)
  Top 0.254: RN8.3 48.71,44.19 v47.9,43.38 46.63,42.11 46.63,41.15 | IC6.32 46.95,38.95 46.63,39.27 46.63,41.15 | 46.63,41.15 43.64,41.15 v43.41,41.38 | IC2.30 32.12,24.25 31.37,23.5 29.46,23.5 29.08,23.88 28.12,23.88 v27.43,23.19 | JP1.3 36.83,49.78 v38.1,48.51
  Bottom 0.254: v47.9,43.38 47.88,43.36 47.88,40.89 48.11,40.66 48.11,33.07 47.7,32.66 39.52,32.66 36.07,29.21 32.69,29.21 31.42,30.48 29.92,30.48 28.4,28.96 28.4,24.16 v27.43,23.19 | v43.41,41.38 43.41,44.35 39.24,48.51 v38.1,48.51
IO11*  (via drill 0.51)
  Top 0.254: 38.85,28.64 IC2.12 38.9,28.57 39.5,28.57 40.01,29.08 43.43,29.08 43.81,29.46 45.97,29.46 46.48,29.97 50.29,29.97 50.67,30.35 50.67,31.5 50.42,31.75 49.91,31.75 47.88,33.78 47.37,33.78 44.58,36.58 42.04,36.58 v41.4,37.21 | JP1.4 34.29,48.54 v34.31,48.51
  Bottom 0.254: v34.31,48.51 32,48.51 31.11,47.62 31.11,44.45 31.7,43.87 33.76,43.87 40.41,37.21 v41.4,37.21
IO12  (via drill 0.51)
  Top 0.254: IC2.26 30.67,26.25 v30.35,25.93
  Bottom 0.254: JP1.5 31.75,50.16 32.61,49.3 39.34,49.3 44.32,44.32 44.32,39.45 44.58,39.19 44.58,36.83 43.81,36.07 37.85,36.07 34.77,33.02 31.37,33.02 30.61,33.66 30.61,36.58 28.57,38.61 26.8,38.61 25.91,37.72 25.91,35.18 24.13,33.4 24.13,22.99 25.65,21.46 29.46,21.46 30.61,22.61 30.61,25.68 v30.35,25.93
IO13*  (via drill 0.51)
  Top 0.254: IC2.32 32.62,23.25 31.14,21.77 v30.99,21.77 29.64,21.77 29.21,21.34 29.21,20.95 28.83,20.57 28.07,20.57 27.61,21.03 IC3.2
  Bottom 0.254: v30.99,21.77 30.18,20.95 25.4,20.95 23.57,22.78 23.57,33.73 25.27,35.43 25.27,37.85 26.54,39.12 28.75,39.12 31.17,36.7 31.17,33.98 31.62,33.53 34.54,33.53 37.72,36.7 38.61,36.7 38.86,36.96 38.86,37.97 33.53,43.31 31.5,43.31 29.21,45.59 JP1.6
LINKLED  (via drill 0.51)
  Top 0.254: IC6.25 47.41,35.43 46.56,35.43 44.7,37.29 44.7,38.81 43.89,39.62 42.29,39.62 41.78,39.12 v41.4,39.12 | LINK.C 28.42,42.39 | T2.3 17.6,48.06 v17.12,48.06 | v27.58,43.54 27.62,43.54 LINK.C | v32.05,44.73 30.84,44.73 LINK.C
  Top 0.305: 28.66,42.42 LINK.C
  Bottom 0.254: v32.05,44.73 33.96,44.73 39.57,39.12 v41.4,39.12 | v27.58,43.54 27.58,43.74 23.27,48.06 v17.12,48.06 14.05,48.06 13.21,48.9 7.87,48.9 3.56,44.58 1.77,44.58 UC1.L4
MISO  (via drill 0.51)
  Top 0.254: v61.85,11.68 62.61,12.45 X2.7 | 47.46,39.98 IC6.34 48.18,39.95 49.99,41.76 v49.99,42.01 | ICSP.1 64.9,31.62 64.9,33.27 63.63,34.54 63.63,36.83 65.02,38.23 65.02,44.58 63.88,45.72 60.33,45.72 v59.94,46.1 | IC2.11 39.81,27.75 40.64,28.57 42.29,28.57 42.67,28.19 43.94,28.19 v44.27,28.52
  Bottom 0.254: v44.27,28.52 44.27,29.79 45.47,30.99 49.28,30.99 49.99,31.7 v49.99,42.01 49.99,42.37 50.93,43.31 50.93,43.81 51.44,44.32 52.7,44.32 53.09,43.94 53.09,43.05 53.47,42.67 59.18,42.67 59.94,43.43 v59.94,46.1
  Bottom 0.305: ICSP.1 65.08,29.16 65.08,24.08 63.63,22.63 63.63,13.08 62.23,11.68 v61.85,11.68
MOSI  (via drill 0.51)
  Top 0.254: IC2.10 40.08,27.25 40.89,28.07 42.04,28.07 42.55,27.56 44.83,27.56 v45.72,28.45 | IC10.2 51.69,18.31 51.92,18.54 51.92,19.1 52.38,19.56 53.47,19.56 54.43,20.52 v54.43,21.74 54.43,22.66 52.96,24.13 52.17,24.13 51.28,25.02 51.28,26.29 v51.23,26.34
  Top 0.305: ICSP.4 65.02,29.21 63.04,29.21 60.4,26.57 v60.4,25.7
  Bottom 0.254: v51.23,26.34 50.65,26.92 49.78,26.92 47.88,25.02 46.86,25.02 46.35,25.53 46.35,27.18 45.72,27.81 v45.72,28.45
  Bottom 0.305: v60.4,25.7 60.4,22.81 59.31,21.72 54.59,21.72 v54.43,21.74
MOSI3  (via drill 0.51)
  Top 0.254: IC6.35 47.95,40.45 48.51,41.02 48.51,41.78 49.66,42.93 51.18,42.93 51.44,42.67 57.66,42.67 58.42,41.91 58.42,37.31 57.15,36.04 57.15,31.88 57.78,31.24 57.78,27.94 58.67,27.05 58.67,25.02 57.48,23.82 57.48,17.98 v58.18,17.29
  Top 0.305: IC10.4 48.05,18.96 v47.9,18.82 | v61.44,16.87 61.46,16.85 X2.3
  Bottom 0.254: v47.9,18.82 48.17,18.55 56.91,18.55 v58.18,17.29
  Bottom 0.305: v58.18,17.29 61.02,17.29 v61.44,16.87
N$1  (via drill 0.51)
  Top 0.254: v5.69,13.18 5.69,14.96 6.08,15.35 RN1.2 | IC3.4 26.96,18.96 v27.56,18.36
  Bottom 0.254: v5.69,13.18 12.95,21.08 17.91,21.08 18.52,20.47 18.52,19.2 19.05,18.67 27.25,18.67 v27.56,18.36
N$2  (via drill 0.51)
  Top 0.254: 24.86,43.97 RN3.8 24.88,44.05 v24.13,44.76 | RN3.7 26.01,43.05 LINK.A
  Top 0.305: 26.52,42.41 LINK.A | RN3.7 RN3.8
  Bottom 0.305: UC1.L3 3.96,42.14 5.21,40.89 7.52,40.89 12.95,46.33 22.55,46.33 v24.13,44.76
N$3  (via drill 0.51)
  Top 0.254: RN3.5 25.5,41.45 100M.A
  Top 0.305: 26.26,40.81 100M.A 27.08,40.54 27.58,41.05 v27.58,41.45 | RN3.5 RN3.6
  Bottom 0.254: 25.48,42.8 26.82,41.45 v27.58,41.45 | 18.67,42.8 16.26,45.21 13.34,45.21 3.19,35.07 UC1.L1
  Bottom 0.305: 18.67,42.8 25.48,42.8
N$5
  Top 0.305: RN1.7 4.13,15.35 L.A
N$6
  Top 0.254: TX.A 26.17,36.47 R25.1
N$7
  Top 0.254: R25.2 26.59,38.59 RX.A
N$8
  Top 0.305: RN1.8 4.22,14.55 ON.A
N$9
  Top 0.254: ACT.A 26.53,46.31 25.7,47.14 24.88,47.14 RN4.7
  Top 0.305: RN4.7 RN4.8
N$10
  Top 0.254: C1.2 R24.2 17.15,43.23 UC1.R3
N$12
  Top 0.254: IC6.31 48.66,38.45 R14.1 | Q4.1 51.75,41.21 52.2,41.66 54.48,41.66 54.74,41.4 C3.1
  Top 0.305: R14.1 51.37,40.18 Q4.1
N$13
  Top 0.406: ZZ1.P$3 12.38,23.11 13.08,23.11 14.99,25.02 15.24,25.02 16.1,25.88 L10.2
N$14
  Top 0.406: ZZ1.P$4 15.12,23.5 15.12,23.89 16.38,25.15 16.87,25.15 L9.2
N$15
  Top 0.406: ZZ1.P$2 9.83,22.53 11.3,24 12.95,24 14.35,25.4 L8.2
N$16  (via drill 0.51)
  Top 0.406: v12.57,24.89 L7.2
  Bottom 0.406: ZZ1.P$1 6.91,22.66 8.76,24.51 12.19,24.51 v12.57,24.89
N$17
  Top 0.254: 51.61,38.13 52.08,37.66 R1.2
  Top 0.305: 51.61,38.13 Q4.2
N$18
  Top 0.254: Q4.4 53.43,40.25 54.36,39.32 55.31,39.32 R21.1
N$19  (via drill 0.51)
  Top 0.254: 26.04,32.89 C6.2 | 26.06,32.74 C6.2 | C6.2 26.29,32.89 25.15,31.75 23.24,31.75 19.81,28.32 v19.68,28.32
  Top 0.305: UC1.R1 11.81,44.07 9.55,41.81 v9.55,39.62
  Bottom 0.305: v19.68,28.32 19.3,28.7 11.68,28.7 11.3,28.96 11.3,31.24 9.53,33.02 9.53,39.6 v9.55,39.62
N$20
  Top 0.254: RN9.4 45.55,44.53 44.91,43.89 IC6.39
N$21
  Top 0.254: R23.1 R22.1 C4.2
N$22  (via drill 0.51)
  Top 0.254: v21.72,36.83 21.72,36.7 22.1,36.32 22.99,36.32 C7.2
  Bottom 0.254: v21.72,36.83 21.72,40.26 20.7,41.27 18.67,41.27 17.14,39.75 17.14,38.35 16.64,37.85 14.73,37.85 13.46,36.58 11.94,36.58 10.79,37.72 10.79,41.53 12.06,42.8 UC1.R2
N$24
  Top 0.254: 49.33,30.63 49.33,31.29 47.47,33.15 45.7,33.15 45.41,33.44 IC6.23
  Top 0.305: 49.33,30.63 R2.2
N$25
  Top 0.254: R5.1 R6.2 25.15,13.06 25.15,9.27 25.37,9.04 IC5.1
N$26
  Top 0.254: IC4.1 11.89,18.36 11.68,18.16 10.67,18.16 10.29,17.78 10.29,15.49 9.4,14.61 R29.2 R28.1
N$27
  Top 0.229: IC5.17 26.66,10.43 26.42,10.67
  Top 0.254: 26.42,10.67 26.42,11.56 R7.2
N$28
  Top 0.254: IC4.17 13.14,19.82 13.08,20.14
  Top 0.61: 13.08,20.14 13.08,20.57 R30.2
N$29
  Top 0.254: IC4.18 11.52,19.27 R31.2
N$30
  Top 0.254: RN4.5 24.85,45.59 25.88,44.55 FDX.A
  Top 0.305: RN4.5 RN4.6 | 26.48,44.09 FDX.A
N$31
  Top 0.254: RN9.3 44.75,44.42 44.4,44.07 IC6.40
N$32
  Top 0.305: R9.1 18.09,22.02 ZZ1.P$5
N$33
  Top 0.305: R9.2 19.86,22.95 ZZ1.P$6
N$34
  Top 0.305: R8.2 R10.1 55.05,27.75 ZZ1.P$9
N$35
  Top 0.254: 43.92,45.17 RN9.2 43.91,45.15 IC6.41
N$36
  Top 0.254: IC5.18 25.65,10.45 25.65,11.94 26.04,12.32 28.07,12.32 R32.2
N$37
  Top 0.254: RN9.1 43.15,44.33 43.41,44.07 IC6.42
N$38
  Top 0.254: IC6.20 43.91,32.8 44.83,31.88 44.83,31.07 C46.+
N$39
  Top 0.254: RN8.1 46.87,44.91 46.58,44.91 45.41,43.73 IC6.38
N$40
  Top 0.254: IC6.10 37.59,36.45 R3.2
OSC2E1
  Top 0.254: IC6.30 49.94,37.95 R14.2 50.39,39.09 50.57,39.27 52.58,39.27 53.55,38.29 Q4.3
  Top 0.305: 53.43,38.42 Q4.3 54.73,38.14 C5.1
PMODE0
  Top 0.254: 35.51,44.81 36.17,44.15 38.61,44.15 39.29,43.46 41.53,43.46 41.91,43.08 IC6.45
  Top 0.305: R11.2 R4.1 35.51,44.81
PMODE1
  Top 0.254: 38.86,44.81 39.62,44.04 41.91,44.04 42.41,43.55 IC6.44
  Top 0.305: R15.2 R12.1 38.86,44.81
PMODE2
  Top 0.254: 41.96,44.76 42.91,43.81 IC6.43
  Top 0.305: R20.2 R19.1 41.96,44.76
RD+  (via drill 0.51)
  Top 0.254: IC2.4 40.15,24.25 40.54,24.64 41.38,24.64 v41.88,24.13 | v8.23,28.02 R27.2
  Bottom 0.254: v8.23,28.02 8.69,27.56 17.78,27.56 21.72,23.62 21.72,22.99 22.73,21.97 22.73,21.01 23.24,20.5 30.89,20.5 34.77,24.38 41.63,24.38 v41.88,24.13
RD-  (via drill 0.51)
  Top 0.254: v6.71,28.09 R26.2 | IC2.3 40.67,23.75 v40.82,23.6
  Bottom 0.254: v6.71,28.09 6.71,27.58 7.24,27.05 17.53,27.05 21.21,23.37 21.21,22.73 22.23,21.72 22.23,20.83 23.11,19.94 31.17,19.94 35,23.77 40.64,23.77 v40.82,23.6
RESET  (via drill 0.51)
  Top 0.254: RESET.1 RESET.2 | ICSP.5 63.5,25.4 61.59,23.5 v58.42,23.5 | IC2.13 38.35,28.95 38.63,29.23 39.4,29.23 40.03,29.87 v40.03,30.84 | v39.5,13.66 39.5,11.43 38.51,10.44 32.92,10.44 32.38,9.91 32.38,6.86 33.02,6.22 v34.29,6.22
  Top 0.305: v1.37,32 1.37,32.23 3.3,34.16 3.3,40.13 4.57,41.4 4.57,42.67 3.43,43.81 3.43,45.47 2.79,46.1 1.52,46.1 1.02,46.61 1.02,51.18 1.91,52.07 3,52.07 RESET.1 | JP3.3 31.5,1.02 23.11,1.02 21.59,2.54 v21.59,3.3 | v54.3,43.48 58.12,43.48 59.82,41.78 59.82,41.48 D4.A
  Top 0.406: R16.1 60.33,40.97 D4.A | IC1.3 54.31,43.7 v54.3,43.48
  Bottom 0.254: 44.2,27.58 44.2,24.64 46.18,22.66 46.18,20.02 45.34,19.18 45.34,18.54 | v58.42,23.5 52.32,23.5 51.18,22.35 48.9,22.35 47.88,23.37 47.12,23.37 45.85,24.64 45.85,26.92 45.19,27.58 44.2,27.58 | 54.3,44.33 53.68,44.96 51.18,44.96 50.16,43.94 50.16,43.56 49.02,42.42 49.02,41.27 49.38,40.92 49.38,32.26 48.67,31.55 40.74,31.55 v40.03,30.84 40.03,28.3 40.39,28.07 42.04,28.07 42.52,27.58 44.2,27.58 | 54.3,44.33 54.31,44.32 | v54.3,43.48 54.3,44.33
  Bottom 0.305: v1.37,32 1.37,31.29 1.91,30.76 4.45,30.76 5.33,29.87 5.33,24.26 4.57,23.5 4.57,21.34 5.23,20.68 5.23,17.42 3.68,15.88 3.68,11.94 4.32,11.3 12.83,11.3 14.86,9.27 14.86,5.97 17.53,3.3 v21.59,3.3 | JP3.3 33.02,4.95 v34.29,6.22 | 45.34,18.54 43.69,17.02 38.99,17.02 38.23,16.13 38.23,14.94 v39.5,13.66
RESET_W
  Top 0.254: 47.9,45.14 47.9,44.6 47.7,44.4 46.79,44.4 45.91,43.52 IC6.37 | RN8.2 47.91,45.5 48.28,45.87 50.04,45.87 51.04,44.87 IC1.2 52.1,44.86
  Top 0.305: 47.9,45.14 RN8.2
RXIN  (via drill 0.51)
  Top 0.254: IC6.5 37.91,38.95 37.24,39.62 32.18,39.62 v32.03,39.47 | R22.2 23.01,34.54 v23.88,35.41 24.79,36.32 C7.1
  Bottom 0.254: v23.88,35.41 24.69,36.22 24.69,38 26.26,39.62 28.93,39.62 29.72,38.84 30.33,38.84 30.99,39.5 32,39.5 v32.03,39.47
RXIP
  Top 0.254: IC6.6 38.96,38.45 38.96,38.46 37.72,38.46 37.06,39.12 32.97,39.12 31.75,37.9 31.75,34.54 31.11,33.91 31.11,31.62 30.61,31.11 28.57,31.11 27.94,31.75 27.94,32.87 C6.1
  Top 0.305: R23.2 C6.1
RXLED  (via drill 0.51)
  Top 0.254: IC2.8 40.95,26.25 v41.43,26.72 | RX.C 28.6,38.53 v27.58,37.52
  Bottom 0.254: v41.43,26.72 38.76,26.72 37.49,27.99 32.56,27.99 31.22,29.34 30.23,29.34 29.46,28.57 29.46,24 30.1,23.37 30.1,22.86 29.34,22.1 25.78,22.1 24.77,23.11 24.77,33.15 26.54,34.92 26.54,36.47 v27.58,37.52
SCK  (via drill 0.51)
  Top 0.254: IC2.9 40.34,26.75 41.15,27.56 41.78,27.56 42.29,27.05 44.6,27.05 v45.03,26.62
  Top 0.305: IC11.2 v52.63,15.44 | ICSP.3 64.97,26.72 64.97,24.46 64.69,24.18 63.04,24.18 61.85,22.99 59.18,22.99 58.17,21.97 58.17,18.54 59.05,17.65 59.05,15.11 v58.67,14.73
  Bottom 0.254: 52.58,15.39 46.53,15.39 45.85,16.08 45.85,18.92 46.79,19.86 46.79,22.86 44.7,24.94 44.7,26.29 v45.03,26.62
  Bottom 0.305: 52.58,15.39 v52.63,15.44 56.41,15.42 57.12,14.71 v58.67,14.73
SCK3  (via drill 0.51)
  Top 0.254: IC6.33 47.46,39.42 48.31,39.42 50.04,41.15 50.55,41.15 51.56,42.16 57.4,42.16 57.91,41.66 57.91,37.47 56.64,36.2 56.64,31.62 57.28,30.99 57.28,27.91 56.34,26.98 56.34,24.56 57.02,23.88 57.02,17.55 v56.77,17.3
  Top 0.305: 63.5,14.61 X2.5 | 63.47,14.68 X2.5 | IC11.4 48.68,16.09 v47.9,16.87 | v61.42,14.71 61.47,14.65 X2.5
  Bottom 0.305: v61.42,14.71 59.77,16.36 57.05,16.36 56.77,16.64 | 56.77,16.64 v56.77,17.3 | v47.9,16.87 54,16.87 54.23,16.64 56.77,16.64
SEN3  (via drill 0.51)
  Top 0.254: IC12.4 48.48,23.26 v47.65,22.43
  Top 0.305: v61.44,18.24 61.73,17.95 X2.2
  Bottom 0.305: v61.44,18.24 58.04,18.24 57.15,19.13 50.72,19.13 47.65,22.2 v47.65,22.43
SPDLED  (via drill 0.51)
  Top 0.254: IC6.24 45.91,34.51 44.4,36.02 41.15,36.02 40.44,36.73 40.44,40.21 40.13,40.51 40.13,41.15 39.62,41.66 38.99,41.66 37.59,43.05 34.92,43.05 34.67,43.31 31.6,43.31 v29.74,41.45 28.7,40.41 100M.C
  Bottom 0.305: UC1.L2 1.93,34.57 13.1,45.74 16.61,45.74 19.05,43.31 26.29,43.31 27.05,42.55 28.65,42.55 v29.74,41.45
TXLED  (via drill 0.51)
  Top 0.254: 28.63,36.86 TX.C 28.7,36.47 v29.74,35.56 | IC2.22 32.44,28.52 31.24,29.72 26.16,29.72 v25.91,29.97
  Bottom 0.254: v29.74,35.56 29.77,35.41 29.77,33.45 26.29,29.97 v25.91,29.97
TXON  (via drill 0.51)
  Top 0.254: IC6.1 38.91,40.95 37.31,42.55 34.67,42.55 34.42,42.8 32.26,42.8 30.07,40.62 v30.07,39.73 | RN2.7 18.33,40.26 UC1.R4
  Bottom 0.254: UC1.R4 16.13,40.26 17.65,41.78 25.02,41.78 26.67,40.13 29.67,40.13 v30.07,39.73
TXOP  (via drill 0.51)
  Top 0.254: IC6.2 38.39,40.45 36.8,42.04 34.42,42.04 34.16,42.29 32.77,42.29 31.22,40.74 v31.22,40.34 | RN2.8 16.03,39.57 UC1.R5
  Bottom 0.254: v31.22,40.34 30.91,40.64 26.92,40.64 25.27,42.29 17.14,42.29 16.64,42.8 14.61,42.8 13.34,41.53 11.94,41.53 11.56,41.15 11.56,39.37 11.94,38.99 UC1.R5
UCAP
  Top 0.254: IC2.6 42.32,25.25 43.76,23.8 44.6,23.8 C25.1
USHIELD
  Top 0.254: USB1.P$2 USB1.S3
  pour Top (isolate 0.305): 0.05,30.38 5.54,30.38 5.49,26.21 3.66,26.21 3.66,18.11 0.05,18.11
  pour Bottom (isolate 0.305): 0.91,30.07 4.17,30.07 4.17,17.98 0.81,17.98
V1+
  Top 0.305: 12.95,32.68 UC1.R10
  Top 0.406: L7.1 12.57,32.3 UC1.R10 | 12.95,32.68 12.95,33.27 14.86,35.18 16.26,35.18 16.76,35.69 C9.2
V1-
  Top 0.406: L8.1 14.35,30.86 15.45,31.96 UC1.R9 17.85,33.91 C12.2
V2+  (via drill 0.51)
  Top 0.305: v17.78,30.1 17.78,28.56 L9.1
  Top 0.406: C29.2 16.67,37.67 UC1.R7
  Bottom 0.305: UC1.R7 15.62,36.45
  Bottom 0.406: 15.62,36.45 17.14,34.92 17.14,30.73 v17.78,30.1
V2-  (via drill 0.51)
  Top 0.305: 16.13,28.3 L10.1
  Top 0.406: L10.1 v16.13,30.1 16.13,30.73 17.12,31.73 C23.2
  Bottom 0.406: UC1.R8 12.91,34.46 16.13,31.24 v16.13,30.1
VIN  (via drill 0.51, 0.81)
  Top 0.229: IC5.16 27.16,10.44 | IC4.16 13.64,19.61 13.72,19.82
  Top 0.254: 27.16,10.44 27.84,11.12 | 13.72,19.82 14.22,20.32
  Top 0.305: C15.2 R8.1 52.3,25.76 ZZ1.P$8 55.37,22.69 v55.37,20.07
  Top 0.61: D2.P$1 16.38,9.83 16.89,10.34 v18.49,10.34 | v43.43,12.7 42.28,12.7 C14.+
  Top 0.813: JP3.8 45.72,8.51 v44.07,10.16 44.09,10.19 44.09,11.38 42.53,12.94 C14.+ 42.04,13.72 | v17.48,20.02 16.79,20.7 R30.1 14.61,20.7 14.22,20.32 | T1.2 14.81,13.34 v15.85,13.34 | C11.+ v18.49,10.34 | v29.72,11.68 28.7,11.68 R7.1 28.14,11.43 27.84,11.12
  Bottom 0.254: 29.46,10.29 29.59,10.16 | v55.37,20.07 61.98,20.07 62.99,19.05 62.99,18.16
  Bottom 0.305: 62.99,18.16 62.99,13.59 62.1,12.7 57.66,12.7 56.01,11.05 46.99,11.05 45.34,12.7 v43.43,12.7
  Bottom 0.61: 18.23,10.34 18.59,10.34 18.41,10.16
  Bottom 0.813: 29.59,10.16 26.34,10.16 19.33,17.17 17.53,17.17 17.48,17.22 | v15.85,13.34 15.79,13.55 | v17.48,20.02 17.48,17.22 | v18.49,10.34 18.23,10.34 15.87,12.45 v15.85,13.34 | 29.59,10.16 30.1,9.65 43.56,9.65 v44.07,10.16 | 17.48,17.22 16.66,17.22 15.85,16.41 v15.85,13.34 | 29.59,10.16 29.72,10.29 v29.72,11.68
VIND
  Top 0.813: T1.1 12.47,9.47 JK1.2
VUSB  (via drill 0.51)
  Top 0.254: IC2.7 42.36,25.75 v42.82,26.21 42.82,26.14
  Top 0.305: C32.2 R18.2 9.32,19.43 C31.+ | 9.78,24.93 L5.1 | v18.16,24.38 18.92,24.38 19.43,24.89 19.43,26.8 20.45,27.81 21.84,27.81 23.11,29.08 30.18,29.08 v30.73,28.52 | 9.83,25.2 L5.1 | L5.1 | v10.82,26.09 10.82,25.98 L5.1
  Top 0.406: 42.82,26.14 43.43,25.53 43.43,25.15 44.07,24.51 45.92,24.51 v47.32,25.91 | v7.92,20.34 8.66,20.34 C31.+ | v59,32.38 59.01,33.12 D1.P$2 59.01,35.84 59.72,36.55 D6_NM.A
  Bottom 0.305: v30.73,28.52 31.34,28.52 32.44,27.43 37.13,27.43 38.66,25.91 42.52,25.91 v42.82,26.21 | v7.92,20.34 6.33,20.34 5.08,21.59 5.08,23.24 7.92,26.09 v10.82,26.09 11.15,26.42 16.13,26.42 v18.16,24.38
  Bottom 0.406: v47.32,25.91 47.95,25.91 49.78,27.74 58.12,27.74 58.93,28.8 58.93,32.31 v59,32.38
XTAL1
  Top 0.254: IC2.17 36.35,30.5 R13.1 35.5,31.33 Y1.1
XTAL2
  Top 0.254: IC2.16 36.85,29.61 37.67,30.43 R13.2 37.5,31.11 Y1.3
XUSB
  Top 0.305: USB1.P1 4.67,23.55 5.51,24.38 5.51,25.27 6.2,25.96 8.81,25.96 9.65,26.8 9.65,27.01 L5.2

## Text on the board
Bottom: LEONARDO ETH V1
tPlace: LINK | 100M | Ethernet-V10
tNames: arduino.org | TX | RX | 4 2 | GND | AREF | 3 2 1 0 9 8 | * | * | * | 7 6 5 4 3 2 1 0 | * | * | (*=PWM) | * | 1 1 1 1 | 1 | Arduino | ANALOG IN | RES | 3V3 | 5V Gnd 12V | 0 1 2 3 4 5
